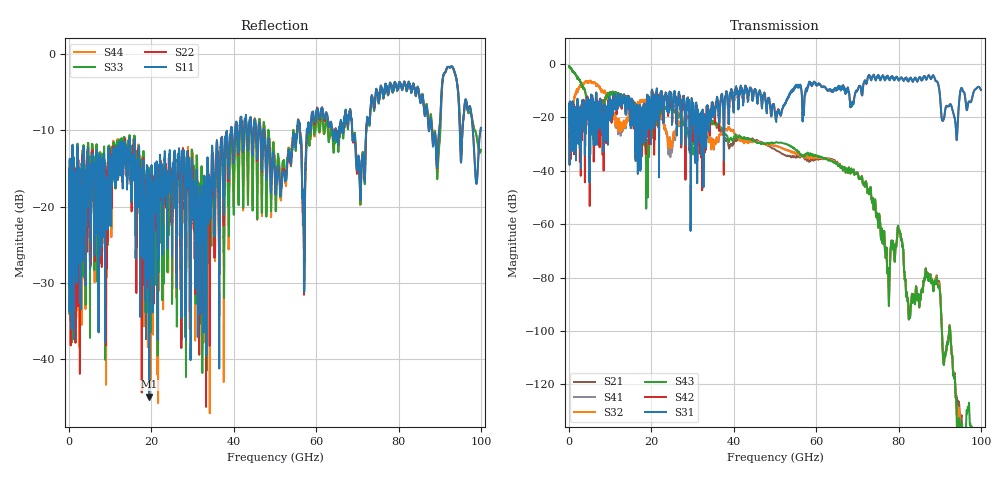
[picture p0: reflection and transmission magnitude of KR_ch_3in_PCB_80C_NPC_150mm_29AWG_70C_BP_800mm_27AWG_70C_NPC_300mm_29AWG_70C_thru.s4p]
# GHz S RI R 45
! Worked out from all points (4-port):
!   4000 points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, 25 MHz to 100 GHz, reference 45 ohm
!   strongest paths, dB at 25 MHz, 25.02 GHz, 50.02 GHz, 75.03 GHz, 100 GHz:
!     S31: -20.7, -20.7, -18.9, -4.2, -9.7
!     S42: -20.7, -17.7, -18.0, -4.4, -9.7
!     S43: -0.8, -16.5, -29.5, -59.4, -151.1
!     S32: -35.7, -30.4, -30.7, -59.4, -157.6
!     S41: -35.7, -32.8, -30.6, -59.4, -157.9
!     S21: -0.9, -16.4, -32.1, -59.5, -168.3
!   lowest |S11| = -44.9 dB at 19.5 GHz (marker M1), VSWR 1.01, Z = 45.3 - j0.441 ohm
!   |S11| at or under -10 dB: start of sweep to 39.34 GHz; 47.31 GHz to 55.46 GHz (8.147 GHz wide, 15.9 % of centre); 68.75 GHz to 72.18 GHz (3.437 GHz wide, 4.88 % of centre)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
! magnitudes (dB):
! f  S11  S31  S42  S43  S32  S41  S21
! 25 MHz  -16.4  -20.7  -20.7  -0.8  -35.7  -35.7  -0.9
! 3.825 GHz  -17.4  -28.6  -22.5  -9.8  -6.8  -6.9  -9.9
! 19.5 GHz  -44.9  -14.6  -30.3  -28.9  -14.5  -14.6  -24.0
! 63.6 GHz  -8.9  -10.2  -9.7  -36.5  -36.1  -36.2  -35.8
! 73.03 GHz  -8.7  -4.7  -4.5  -48.3  -48.3  -48.3  -48.4
! 77.47 GHz  -5.2  -5.1  -4.7  -78.3  -78.4  -78.4  -78.4
! 100 GHz  -9.7  -9.7  -9.7  -151.1  -157.6  -157.9  -168.3
